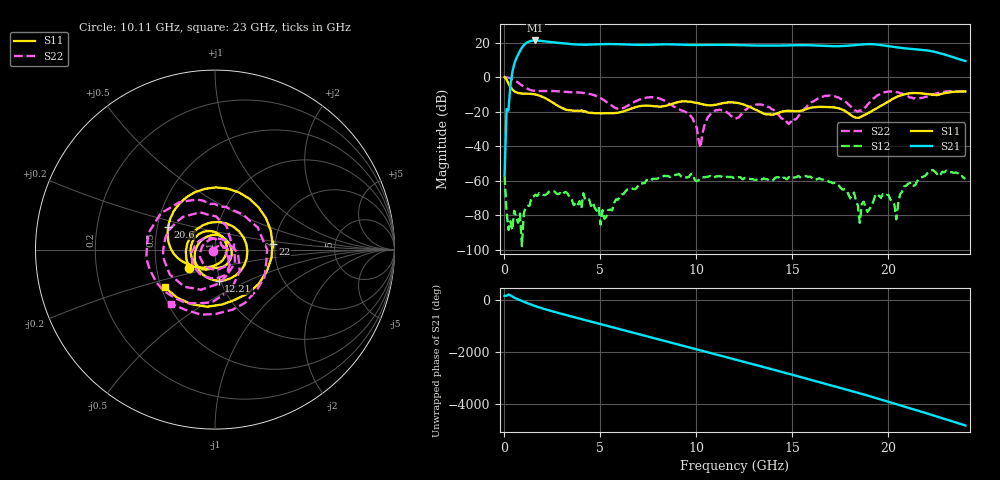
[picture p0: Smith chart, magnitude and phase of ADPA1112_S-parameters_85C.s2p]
! Analog Devices Inc.
! Device:  ADPA1112
! Description: 15 W, GaN Power Amplifier
! Frequency:  1 GHz to 22 GHz
! Package:
! Conditions:	Vdd = 28.0 V
!		Idd = 600 mA
!		Temp = +85 C
! The board loss has been subtracted from S21 Magnitude. Reference for all other parameters are at the connectors.
! Misc:JB
! Note: Analog Devices supplies this data as a sample of measured data for this product.
! Your particular data for this product may vary.
! Analog Devices reserves the right to change this data at anytime
! Freq(GHz)	S11a(dB)	S11p(deg)	S21a(dB)	S21p(deg)	S12a(dB)	S12p(deg)	S22a(dB)	S22p(deg)
# GHz S  dB  R 50
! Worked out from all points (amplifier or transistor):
!   241 points, 10 MHz to 24 GHz, reference 50 ohm
!   highest |S21| = 21.2 dB at 1.61 GHz (marker M1)
!   |S21| within 3 dB of that: 991.9 MHz to 13.73 GHz (12.74 GHz wide, 173 % of centre)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
!   unconditionally stable (mu >= 1): 33.28 MHz to end of sweep
!   at 4.009 GHz: K = 316.99, MAG = 19.4 dB, |S12| = -76.1 dB
!   at 12.01 GHz: K = 44.91, MAG = 18.7 dB, |S12| = -58.0 dB
!   at 24 GHz: K = 110.67, MAG = 10.7 dB, |S12| = -58.9 dB
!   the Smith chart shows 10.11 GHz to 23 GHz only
!   S11 on the Smith chart (normalised r, x): 10.11 GHz: 0.74, -0.15; 12.21 GHz: 0.98, -0.35; 20.6 GHz: 0.57, +0.16; 22 GHz: 1.94, +0.13; 23 GHz: 0.52, -0.25
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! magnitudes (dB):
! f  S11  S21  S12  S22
! 10 MHz  0.0  -56.9  -57.4  0.0
! 110 MHz  -1.5  -18.6  -77.3  -0.2
! 409.9 MHz  -7.2  2.8  -88.6  -1.2
! 1.61 GHz  -10.0  21.2  -68.1  -8.0
! 4.009 GHz  -19.3  18.8  -76.1  -9.0
! 5.309 GHz  -20.9  19.2  -80.9  -14.4
! 8.108 GHz  -17.1  18.9  -58.0  -12.5
! 10.11 GHz  -15.2  18.6  -59.8  -36.3
! 10.81 GHz  -16.3  18.7  -57.9  -20.4
! 12.01 GHz  -14.8  18.6  -58.0  -24.1
! 12.21 GHz  -15.1  18.5  -58.0  -23.4
! 13.41 GHz  -20.7  18.3  -59.3  -15.9
! 14.81 GHz  -19.5  18.4  -57.9  -27.2
! 16.01 GHz  -17.6  18.4  -58.3  -14.4
! 18.21 GHz  -23.1  18.5  -66.9  -19.2
! 18.51 GHz  -23.4  18.8  -84.4  -19.2
! 20.1 GHz  -13.4  17.8  -71.2  -8.3
! 20.4 GHz  -11.6  17.3  -82.4  -8.7
! 20.6 GHz  -10.7  17.0  -67.9  -9.3
! 22 GHz  -9.8  15.4  -56.0  -11.4
! 23 GHz  -9.1  12.8  -54.3  -8.2
! 24 GHz  -8.3  9.3  -58.9  -8.5
